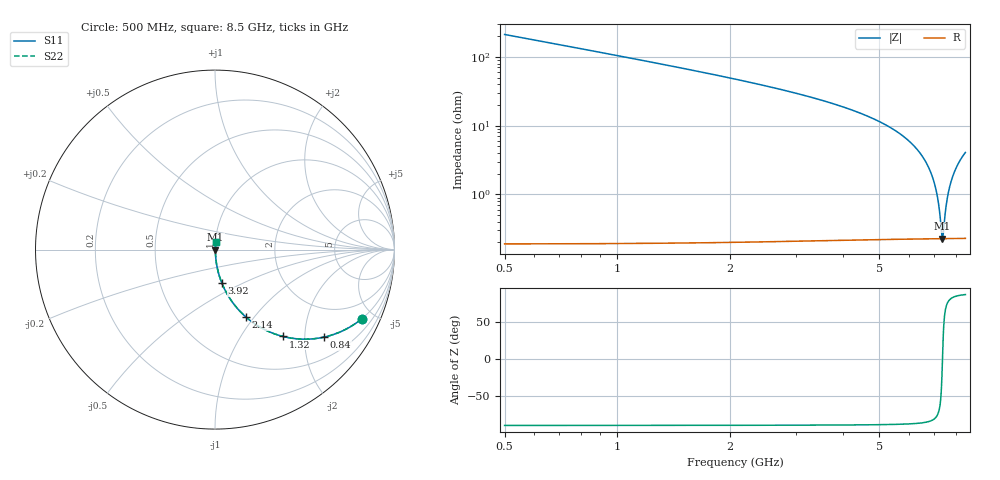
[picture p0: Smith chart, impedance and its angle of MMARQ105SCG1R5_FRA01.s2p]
! MMARQ105SCG1R5_FRA01  S-PARAMETER MODEL  ( General Type )
! Model Generated by TAIYO YUDEN Corporation (http://www.ty-top.com)
! Version 1.0
! TAIYO YUDEN Control No. 200326
! Copyright(c) 2020 TAIYO YUDEN CO.,LTD. All Rights Reserved.
! Product Description (link to TY-COMPAS)
! https://ds.yuden.co.jp/TYCOMPAS/or/detail?pn=MMARQ105SCG1R5BFRA01&u=M
! Products Name : Multilayer Ceramic Capacitors
! Characteristics :
!  Capacitance : 1.5 pF , Rated Voltage : 250V , TCC : CG / C0G
!  Case Size : 1.0 x 0.5 / 0.039 x 0.02 [mm/inch] , Thickness : 0.5 / 0.02 [mm/inch]
!  (Conditions: Temperature = 25 degC , DC Bias Current/Voltage = 0A / 0V)
! External Node Assignments :
!  1  o---| |---o  2
! GND o---------o GND
! Frequency Range : 500MHz  -  8.5GHz  [ 401 STEP ]
# MHz S RI R 50
! Freq[MHz].  S11 Real  S11 Imag  S21 Real  S21 Imag  S12 Real  S12 Imag  S22 Real  S22 Imag
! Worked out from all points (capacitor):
!   401 points, 500 MHz to 8.5 GHz, reference 50 ohm
!   read as one part in series: C = 1.5 pF near 540 MHz
!   lowest |Z| = 227 mohm at 7.38 GHz (marker M1)
!   series resonance near 7.383 GHz, so ESL is about 310 pH
!   S11 on the Smith chart (normalised r, x): 500 MHz: 1.00, -4.23; 840 MHz: 1.00, -2.50; 1.32 GHz: 1.00, -1.56; 2.14 GHz: 1.00, -0.91; 3.92 GHz: 1.00, -0.39; 8.5 GHz: 1.00, +0.08
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500  0.8171 -0.3861  0.1829 0.3861  0.1829 0.3861  0.8171 -0.3861
840  0.609 -0.4872  0.391 0.4872  0.391 0.4872  0.609 -0.4872
1320  0.378 -0.4836  0.622 0.4836  0.622 0.4836  0.378 -0.4836
1840  0.2275 -0.4174  0.7725 0.4174  0.7725 0.4174  0.2275 -0.4174
2140  0.1724 -0.3755  0.8276 0.3755  0.8276 0.3755  0.1724 -0.3755
3180  0.0706 -0.2523  0.9294 0.2523  0.9294 0.2523  0.0706 -0.2523
3920  0.0384 -0.1866  0.9616 0.1866  0.9616 0.1866  0.0384 -0.1866
4500  0.0235 -0.1445  0.9765 0.1445  0.9765 0.1445  0.0235 -0.1445
5840  0.0068 -0.0674  0.9932 0.0674  0.9932 0.0674  0.0068 -0.0674
6340  0.00416 -0.0437  0.9958 0.0437  0.9958 0.0437  0.00416 -0.0437
6720  0.00298 -0.027  0.997 0.027  0.997 0.027  0.00298 -0.027
7000  0.00249 -0.0153  0.9975 0.0153  0.9975 0.0153  0.00249 -0.0153
7180  0.00232 -0.00799  0.9977 0.00799  0.9977 0.00799  0.00232 -0.00799
7260  0.00229 -0.00482  0.9977 0.00482  0.9977 0.00482  0.00229 -0.00482
7340  0.00227 -0.00168  0.9977 0.00168  0.9977 0.00168  0.00227 -0.00168
7380  0.00226 -0.000126  0.9977 0.000126  0.9977 0.000126  0.00226 -0.000126
7420  0.00227 0.00142  0.9977 -0.00142  0.9977 -0.00142  0.00227 0.00142
7520  0.00229 0.00525  0.9977 -0.00525  0.9977 -0.00525  0.00229 0.00525
7580  0.00232 0.00753  0.9977 -0.00753  0.9977 -0.00753  0.00232 0.00753
7760  0.00247 0.0142  0.9975 -0.0142  0.9975 -0.0142  0.00247 0.0142
8080  0.00295 0.0258  0.9971 -0.0258  0.9971 -0.0258  0.00295 0.0258
8500  0.00392 0.0404  0.9961 -0.0404  0.9961 -0.0404  0.00392 0.0404
